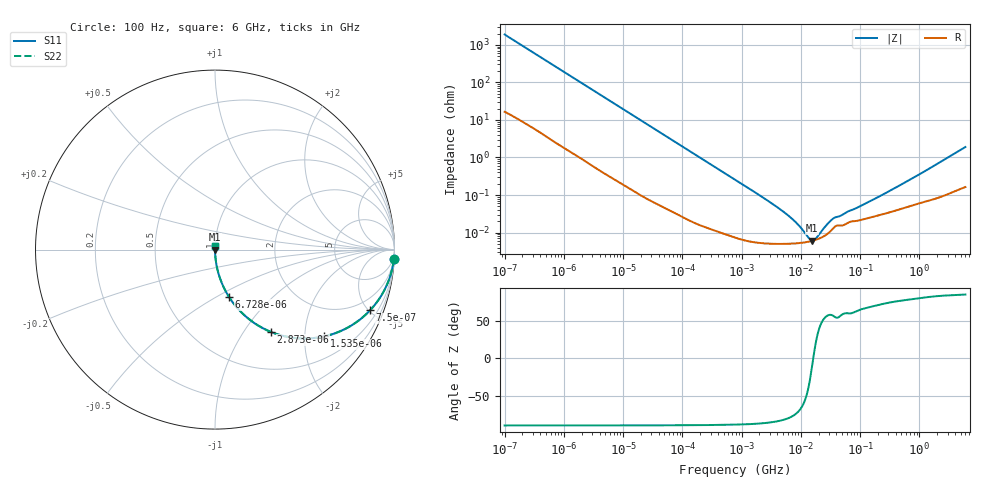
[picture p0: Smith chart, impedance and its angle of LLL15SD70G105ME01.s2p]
!Murata Part Number: LLL15SD70G105ME01
!These Parameters are Measured in Series Mode Connection
!Data Generated on Mar 13, 2026
!  o--ll--o
!Port1  Port2
!  o------o
!Operation Temp=25[degC], DC Bias Voltage=0[V]
!Freq. Start=100[Hz] Stop=6[GHz] 401[Steps]
# Hz S RI R 50
!Freq.(Hz) S11(Real) S11(Imag) S21(Real) S21(Imag) S12(Real) S12(Imag) S22(Real) S22(Imag)
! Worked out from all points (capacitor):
!   401 points, 100 Hz to 6 GHz, reference 50 ohm
!   read as one part in series: C = 842 nF near 109 Hz
!   lowest |Z| = 6.1 mohm at 15.56 MHz (marker M1)
!   series resonance near 16.21 MHz, so ESL is about 110 pH
!   S11 on the Smith chart (normalised r, x): 100 Hz: 1, -38; 750 Hz: 1.05, -5.09; 1.535 kHz: 1.02, -2.50; 2.873 kHz: 1.01, -1.34; 6.728 kHz: 1.01, -0.58; 6 GHz: 1.00, +0.04
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100  0.9967 -0.0528  0.00326 0.0528  0.00326 0.0528  0.9967 -0.0528
293  0.9754 -0.1502  0.0246 0.1502  0.0246 0.1502  0.9754 -0.1502
750  0.8642 -0.3379  0.1358 0.3379  0.1358 0.3379  0.8642 -0.3379
1073  0.7589 -0.4231  0.2411 0.4231  0.2411 0.4231  0.7589 -0.4231
1535  0.6087 -0.4833  0.3913 0.4833  0.3913 0.4833  0.6087 -0.4833
2008  0.4782 -0.4948  0.5218 0.4948  0.5218 0.4948  0.4782 -0.4948
2873  0.3117 -0.4585  0.6883 0.4585  0.6883 0.4585  0.3117 -0.4585
4299  0.1701 -0.3711  0.8299 0.3711  0.8299 0.3711  0.1701 -0.3711
6728  0.0786 -0.2643  0.9214 0.2643  0.9214 0.2643  0.0786 -0.2643
15062  0.0176 -0.1267  0.9824 0.1267  0.9824 0.1267  0.0176 -0.1267
40335  0.00288 -0.0483  0.9971 0.0483  0.9971 0.0483  0.00288 -0.0483
774597  7.99e-05 -0.00258  0.9999 0.00258  0.9999 0.00258  7.99e-05 -0.00258
4856642  5.01e-05 -0.000377  0.9999 0.000377  0.9999 0.000377  5.01e-05 -0.000377
7599586  5.12e-05 -0.000206  0.9999 0.000206  0.9999 0.000206  5.12e-05 -0.000206
1.137099e7  5.45e-05 -8.96e-05  0.9999 8.96e-05  0.9999 8.96e-05  5.45e-05 -8.96e-05
1.243624e7  5.58e-05 -6.63e-05  0.9999 6.63e-05  0.9999 6.63e-05  5.58e-05 -6.63e-05
1.555665e7  6.02e-05 -1.01e-05  0.9999 1.01e-05  0.9999 1.01e-05  6.02e-05 -1.01e-05
2.128304e7  7.12e-05 6.78e-05  0.9999 -6.78e-05  0.9999 -6.78e-05  7.12e-05 6.78e-05
3.64232e7  0.000137 0.000203  0.9999 -0.000203  0.9999 -0.000203  0.000137 0.000203
8.918374e7  0.000206 0.000411  0.9998 -0.000411  0.9998 -0.000411  0.000206 0.000411
3.124326e8  0.000345 0.00123  0.9997 -0.00123  0.9997 -0.00123  0.000345 0.00123
6e9  0.00198 0.0189  0.998 -0.0189  0.998 -0.0189  0.00198 0.0189
